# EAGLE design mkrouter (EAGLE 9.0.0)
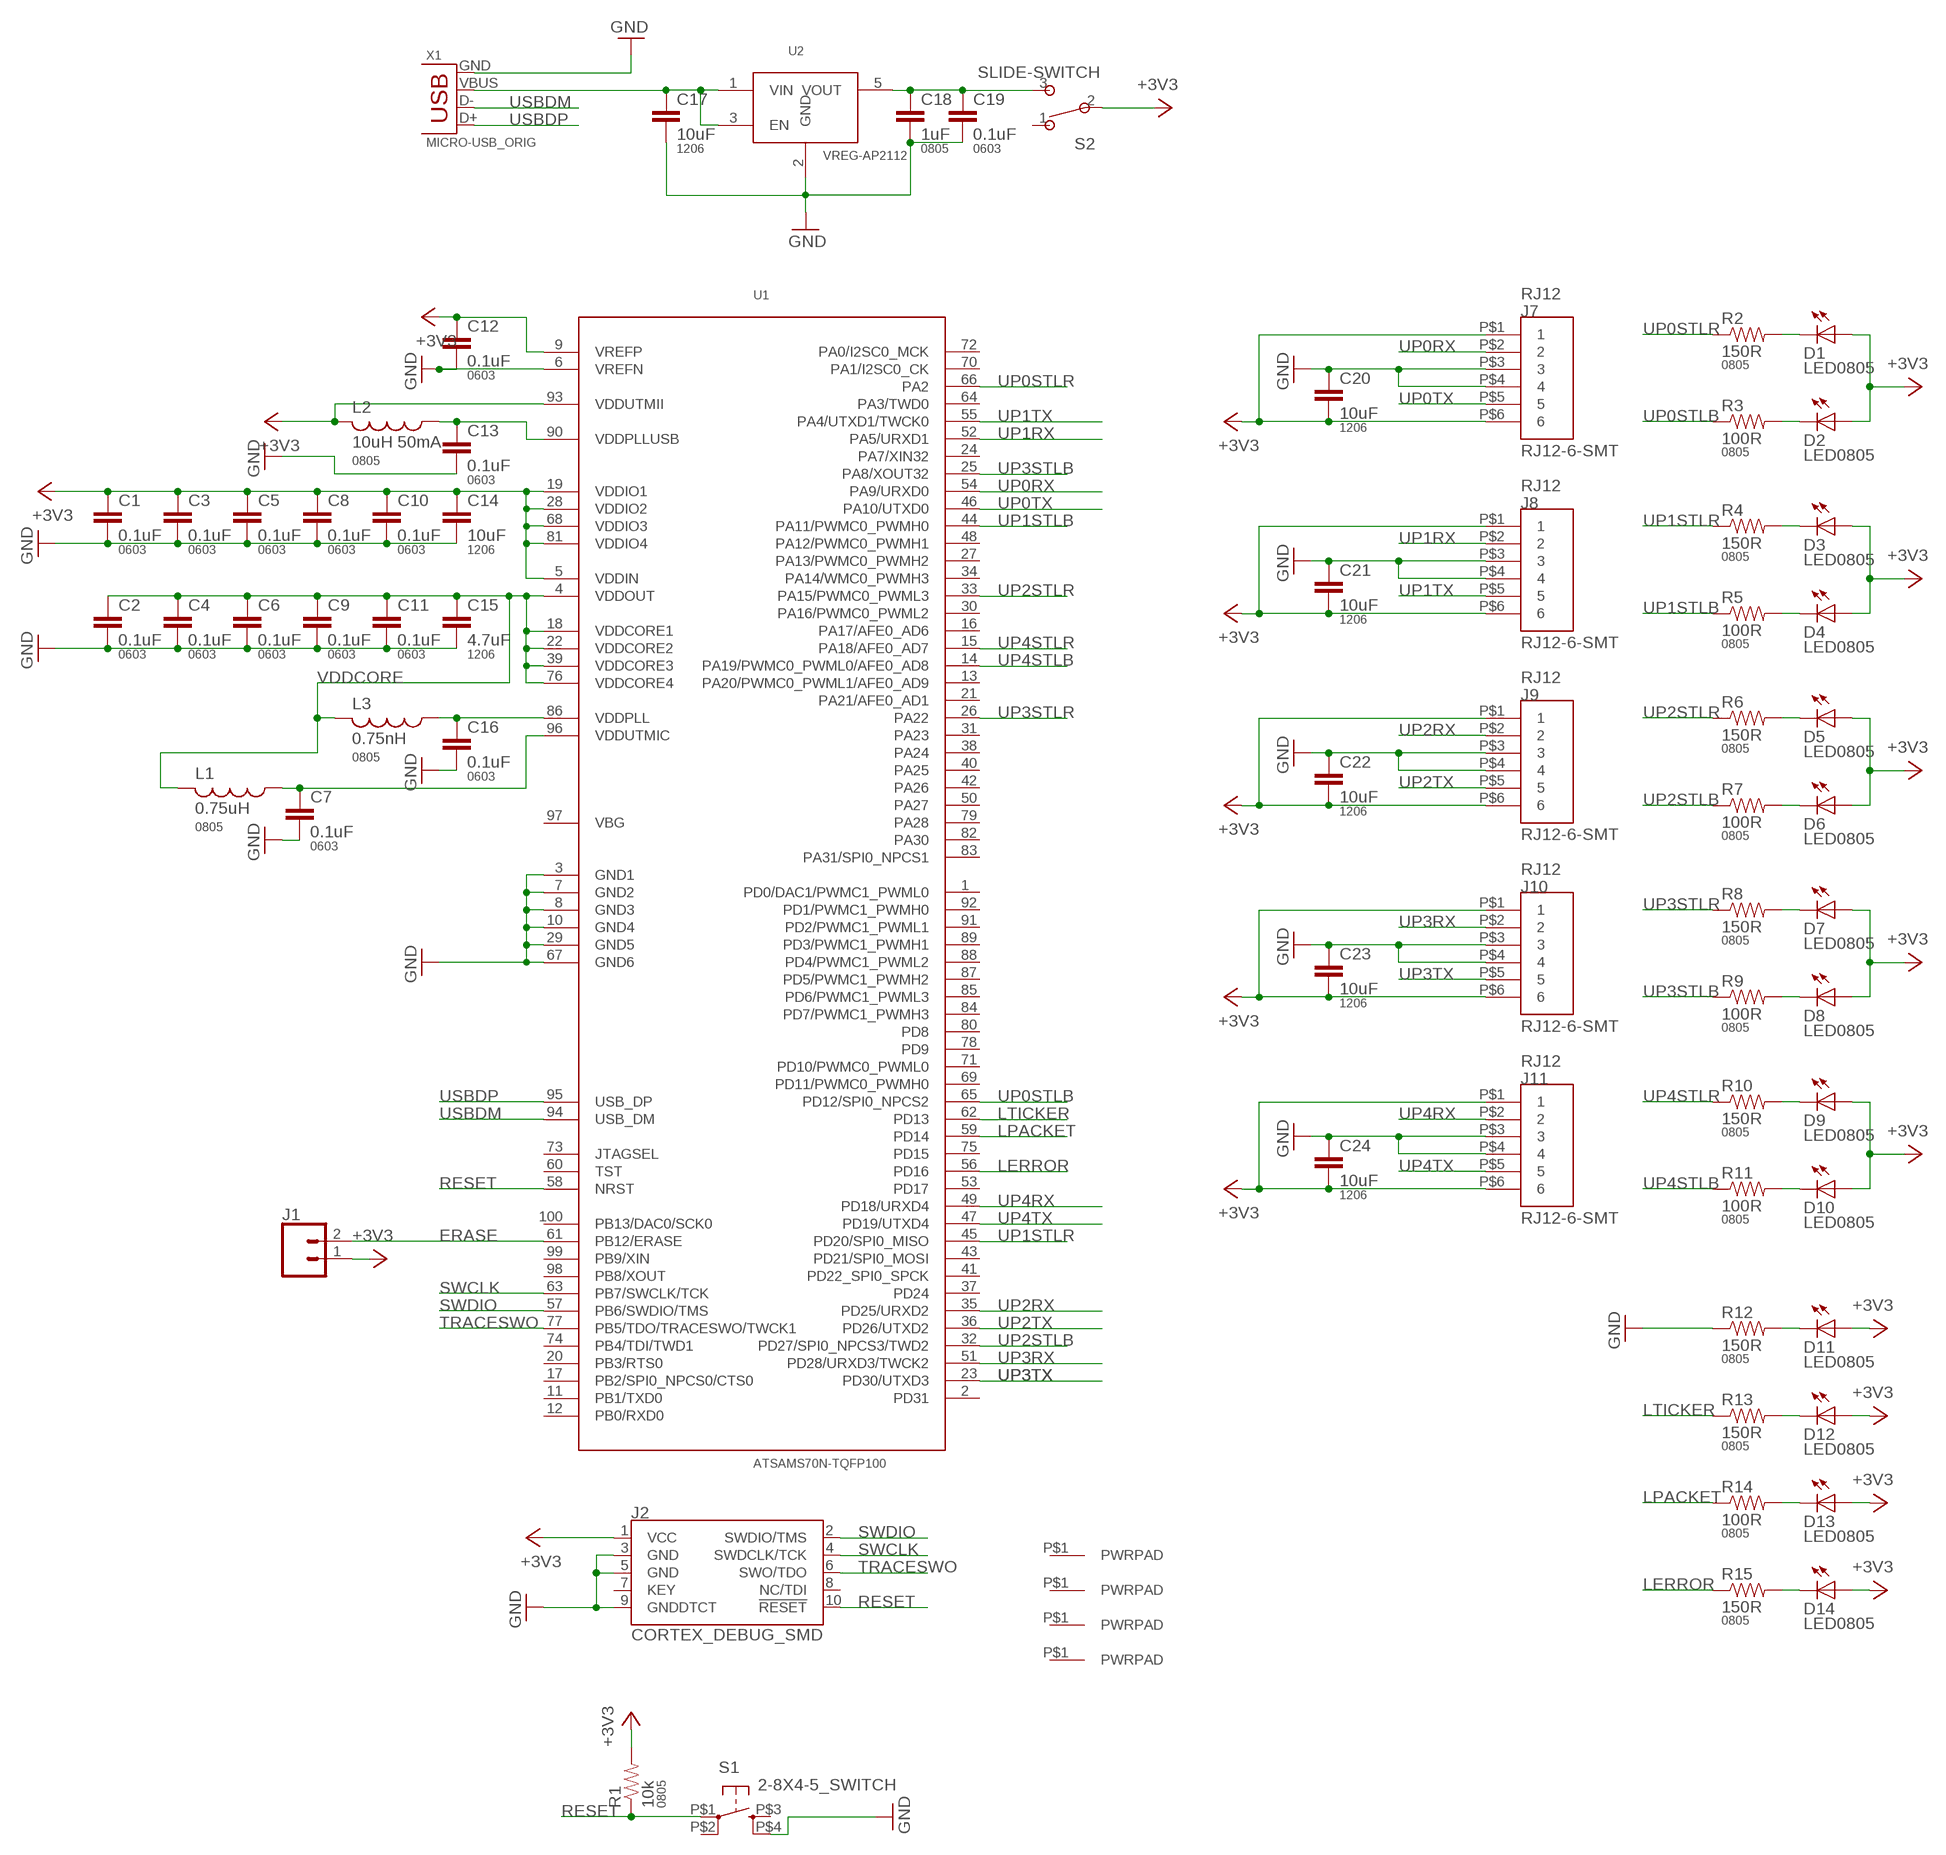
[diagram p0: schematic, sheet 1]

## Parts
C1  0.1uF  CAP0603-CAP  [0603-CAP]
C2  0.1uF  CAP0603-CAP  [0603-CAP]
C3  0.1uF  CAP0603-CAP  [0603-CAP]
C4  0.1uF  CAP0603-CAP  [0603-CAP]
C5  0.1uF  CAP0603-CAP  [0603-CAP]
C6  0.1uF  CAP0603-CAP  [0603-CAP]
C7  0.1uF  CAP0603-CAP  [0603-CAP]
C8  0.1uF  CAP0603-CAP  [0603-CAP]
C9  0.1uF  CAP0603-CAP  [0603-CAP]
C10  0.1uF  CAP0603-CAP  [0603-CAP]
C11  0.1uF  CAP0603-CAP  [0603-CAP]
C12  0.1uF  CAP0603-CAP  [0603-CAP]
C13  0.1uF  CAP0603-CAP  [0603-CAP]
C14  10uF  CAP1206  [1206]
C15  4.7uF  CAP1206  [1206]
C16  0.1uF  CAP0603-CAP  [0603-CAP]
C17  10uF  CAP1206  [1206]
C18  1uF  CAP0805  [0805]
C19  0.1uF  CAP0603-CAP  [0603-CAP]
C20  10uF  CAP1206  [1206]
C21  10uF  CAP1206  [1206]
C22  10uF  CAP1206  [1206]
C23  10uF  CAP1206  [1206]
C24  10uF  CAP1206  [1206]
D1  LED0805  [LED0805]
D2  LED0805  [LED0805]
D3  LED0805  [LED0805]
D4  LED0805  [LED0805]
D5  LED0805  [LED0805]
D6  LED0805  [LED0805]
D7  LED0805  [LED0805]
D8  LED0805  [LED0805]
D9  LED0805  [LED0805]
D10  LED0805  [LED0805]
D11  LED0805  [LED0805]
D12  LED0805  [LED0805]
D13  LED0805  [LED0805]
D14  LED0805  [LED0805]
J1  CONN_021X02_NO_SILK  [1X02_NO_SILK]
J2  CORTEX_DEBUG_SMD  [SAMTECH_FTSH-105-01]
J3  PWRPADM3  [PWRPAD_3-25MM]
J4  PWRPADM3  [PWRPAD_3-25MM]
J5  PWRPADM3  [PWRPAD_3-25MM]
J6  PWRPADM3  [PWRPAD_3-25MM]
J7  RJ12-6-SMT  [RJ12-6-SMT]
J8  RJ12-6-SMT  [RJ12-6-SMT]
J9  RJ12-6-SMT  [RJ12-6-SMT]
J10  RJ12-6-SMT  [RJ12-6-SMT]
J11  RJ12-6-SMT  [RJ12-6-SMT]
L1  0.75uH  INDUCTOR-0805  [0805]
L2  10uH 50mA  INDUCTOR-0805  [0805]
L3  0.75nH  INDUCTOR-0805  [0805]
R1  10k  RESISTOR0805-RES  [0805]
R2  150R  RESISTOR0805-RES  [0805]
R3  100R  RESISTOR0805-RES  [0805]
R4  150R  RESISTOR0805-RES  [0805]
R5  100R  RESISTOR0805-RES  [0805]
R6  150R  RESISTOR0805-RES  [0805]
R7  100R  RESISTOR0805-RES  [0805]
R8  150R  RESISTOR0805-RES  [0805]
R9  100R  RESISTOR0805-RES  [0805]
R10  150R  RESISTOR0805-RES  [0805]
R11  100R  RESISTOR0805-RES  [0805]
R12  150R  RESISTOR0805-RES  [0805]
R13  150R  RESISTOR0805-RES  [0805]
R14  100R  RESISTOR0805-RES  [0805]
R15  150R  RESISTOR0805-RES  [0805]
S1  2-8X4-5_SWITCH  [TACT-SWITCH-KMR6]
S2  SLIDE-SWITCH  [AYZ0102AGRLC]
U1  ATSAMS70N-TQFP100  [TQFP100-14X14]
U2  VREG-AP2112  [SOT23-5]
X1  MICRO-USB_ORIG  [DX4R005HJ5]

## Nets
+3V3: C1.1 C3.1 C5.1 C8.1 C10.1 C12.1 C14.1 C20.2 C21.2 C22.2 C23.2 C24.2 D1.1(A) D2.1(A) D3.1(A) D4.1(A) D5.1(A) D6.1(A) D7.1(A) D8.1(A) D9.1(A) D10.1(A) D11.1(A) D12.1(A) D13.1(A) D14.1(A) J1.1 J2.1(VCC) J7.P$1 J7.P$6 J8.P$1 J8.P$6 J9.P$1 J9.P$6 J10.P$1 J10.P$6 J11.P$1 J11.P$6 L2.2 R1.2 S2.2 U1.5(VDDIN) U1.9(VREFP) U1.19(VDDIO1) U1.28(VDDIO2) U1.68(VDDIO3) U1.81(VDDIO4) U1.93(VDDUTMII)
ERASE: J1.2 U1.61(PB12/ERASE)
GND: C1.2 C2.2 C3.2 C4.2 C5.2 C6.2 C7.2 C8.2 C9.2 C10.2 C11.2 C12.2 C13.2 C14.2 C15.2 C16.2 C17.2 C18.2 C19.2 C20.1 C21.1 C22.1 C23.1 C24.1 J2.3(GND) J2.5(GND) J2.9(GNDDTCT) J7.P$3 J7.P$4 J8.P$3 J8.P$4 J9.P$3 J9.P$4 J10.P$3 J10.P$4 J11.P$3 J11.P$4 R12.1 S1.P$4(S1) U1.3(GND1) U1.6(VREFN) U1.7(GND2) U1.8(GND3) U1.10(GND4) U1.29(GND5) U1.67(GND6) U2.2(GND) X1.GND
LERROR: R15.1 U1.56(PD16)
LPACKET: R14.1 U1.59(PD14)
LTICKER: R13.1 U1.62(PD13)
N$1: C16.1 L3.1 U1.86(VDDPLL)
N$2: D4.2(C) R5.2
N$3: C7.1 L1.1 U1.96(VDDUTMIC)
N$4: C17.1 U2.1(VIN) U2.3(EN) X1.VBUS
N$5: C13.1 L2.1 U1.90(VDDPLLUSB)
N$6: D2.2(C) R3.2
N$7: C18.1 C19.1 S2.3 U2.5(VOUT)
N$8: D1.2(C) R2.2
N$9: D3.2(C) R4.2
N$10: D6.2(C) R7.2
N$11: D5.2(C) R6.2
N$12: D8.2(C) R9.2
N$13: D7.2(C) R8.2
N$14: D10.2(C) R11.2
N$15: D9.2(C) R10.2
N$16: D13.2(C) R14.2
N$17: D14.2(C) R15.2
N$22: D12.2(C) R13.2
N$23: D11.2(C) R12.2
RESET: J2.10(!RESET) R1.1 S1.P$1(P) U1.58(NRST)
SWCLK: J2.4(SWDCLK/TCK) U1.63(PB7/SWCLK/TCK)
SWDIO: J2.2(SWDIO/TMS) U1.57(PB6/SWDIO/TMS)
TRACESWO: J2.6(SWO/TDO) U1.77(PB5/TDO/TRACESWO/TWCK1)
UP0RX: J7.P$2 U1.54(PA9/URXD0)
UP0STLB: R3.1 U1.65(PD12/SPI0_NPCS2)
UP0STLR: R2.1 U1.66(PA2)
UP0TX: J7.P$5 U1.46(PA10/UTXD0)
UP1RX: J8.P$2 U1.52(PA5/URXD1)
UP1STLB: R5.1 U1.44(PA11/PWMC0_PWMH0)
UP1STLR: R4.1 U1.45(PD20/SPI0_MISO)
UP1TX: J8.P$5 U1.55(PA4/UTXD1/TWCK0)
UP2RX: J9.P$2 U1.35(PD25/URXD2)
UP2STLB: R7.1 U1.32(PD27/SPI0_NPCS3/TWD2)
UP2STLR: R6.1 U1.33(PA15/PWMC0_PWML3)
UP2TX: J9.P$5 U1.36(PD26/UTXD2)
UP3RX: J10.P$2 U1.51(PD28/URXD3/TWCK2)
UP3STLB: R9.1 U1.25(PA8/XOUT32)
UP3STLR: R8.1 U1.26(PA22)
UP3TX: J10.P$5 U1.23(PD30/UTXD3)
UP4RX: J11.P$2 U1.49(PD18/URXD4)
UP4STLB: R11.1 U1.14(PA19/PWMC0_PWML0/AFE0_AD8)
UP4STLR: R10.1 U1.15(PA18/AFE0_AD7)
UP4TX: J11.P$5 U1.47(PD19/UTXD4)
USBDM: U1.94(USB_DM) X1.D-
USBDP: U1.95(USB_DP) X1.D+
VDDCORE: C2.1 C4.1 C6.1 C9.1 C11.1 C15.1 L1.2 L3.2 U1.4(VDDOUT) U1.18(VDDCORE1) U1.22(VDDCORE2) U1.39(VDDCORE3) U1.76(VDDCORE4)
Unconnected: J2.7(KEY) J2.8(NC/TDI) J3.P$1(PWRPAD) J4.P$1(PWRPAD) J5.P$1(PWRPAD) J6.P$1(PWRPAD) S1.P$2(P1) S1.P$3(S) S2.1 U1.1(PD0/DAC1/PWMC1_PWML0) U1.2(PD31) U1.11(PB1/TXD0) U1.12(PB0/RXD0) U1.13(PA20/PWMC0_PWML1/AFE0_AD9) U1.16(PA17/AFE0_AD6) U1.17(PB2/SPI0_NPCS0/CTS0) U1.20(PB3/RTS0) U1.21(PA21/AFE0_AD1) U1.24(PA7/XIN32) U1.27(PA13/PWMC0_PWMH2) U1.30(PA16/PWMC0_PWML2) U1.31(PA23) U1.34(PA14/WMC0_PWMH3) U1.37(PD24) U1.38(PA24) U1.40(PA25) U1.41(PD22_SPI0_SPCK) U1.42(PA26) U1.43(PD21/SPI0_MOSI) U1.48(PA12/PWMC0_PWMH1) U1.50(PA27) U1.53(PD17) U1.60(TST) U1.64(PA3/TWD0) U1.69(PD11/PWMC0_PWMH0) U1.70(PA1/I2SC0_CK) U1.71(PD10/PWMC0_PWML0) U1.72(PA0/I2SC0_MCK) U1.73(JTAGSEL) U1.74(PB4/TDI/TWD1) U1.75(PD15) U1.78(PD9) U1.79(PA28) U1.80(PD8) U1.82(PA30) U1.83(PA31/SPI0_NPCS1) U1.84(PD7/PWMC1_PWMH3) U1.85(PD6/PWMC1_PWML3) U1.87(PD5/PWMC1_PWMH2) U1.88(PD4/PWMC1_PWML2) U1.89(PD3/PWMC1_PWMH1) U1.91(PD2/PWMC1_PWML1) U1.92(PD1/PWMC1_PWMH0) U1.97(VBG) U1.98(PB8/XOUT) U1.99(PB9/XIN) U1.100(PB13/DAC0/SCK0)

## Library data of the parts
C1-C13 C16 C19 = borkedlabs-passives:CAP: Capacitor; PACKAGE: 0603
C14 C15 C17 C20-C24 = borkedlabs-passives:CAP: Capacitor; PACKAGE: 1206
C18 = borkedlabs-passives:CAP: Capacitor; PACKAGE: 0805
D1-D14 = lights:LED: LED
J1 = SparkFun-Connectors:CONN_02: Multi connection point. Often used as Generic Header-pin footprint for 0.1 inch spaced/style header connections
J2 = SparkFun-Connectors:CORTEX_DEBUG: Cortex Debug Connector - 10 pin Supports JTAG debug, Serial Wire debug, and Serial Wire Viewer. PTH and SMD connector options available. General Connector Information Products: PTH Connector -via Digi-Key SparkFun PSoc SparkFun T
J3-J6 = power:PWRPAD
J7-J11 = connector:RJ12-6-SMT
L1-L3 = borkedlabs-passives:INDUCTOR; PACKAGE: 0805
R1-R15 = borkedlabs-passives:RESISTOR: Resistor; PACKAGE: 0805
S1 = fab:2-8X4-5_SWITCH
S2 = fab:SLIDE-SWITCH: SMD slide-switch AYZ0102AGRLC as found in the fablab inventory. Includes the mounting holes. Made by Zaerc.
U1 = atsam:ATSAMS70N-TQFP100
U2 = power:VREG-AP2112
X1 = fab:MICRO-USB: SMD micro USB connector as found in the fablab inventory. Three footprint variants included: original, as described by manufacturer's datasheet for milling with the 1/100" bit for milling with the 1/64" bit Made by Zaerc.

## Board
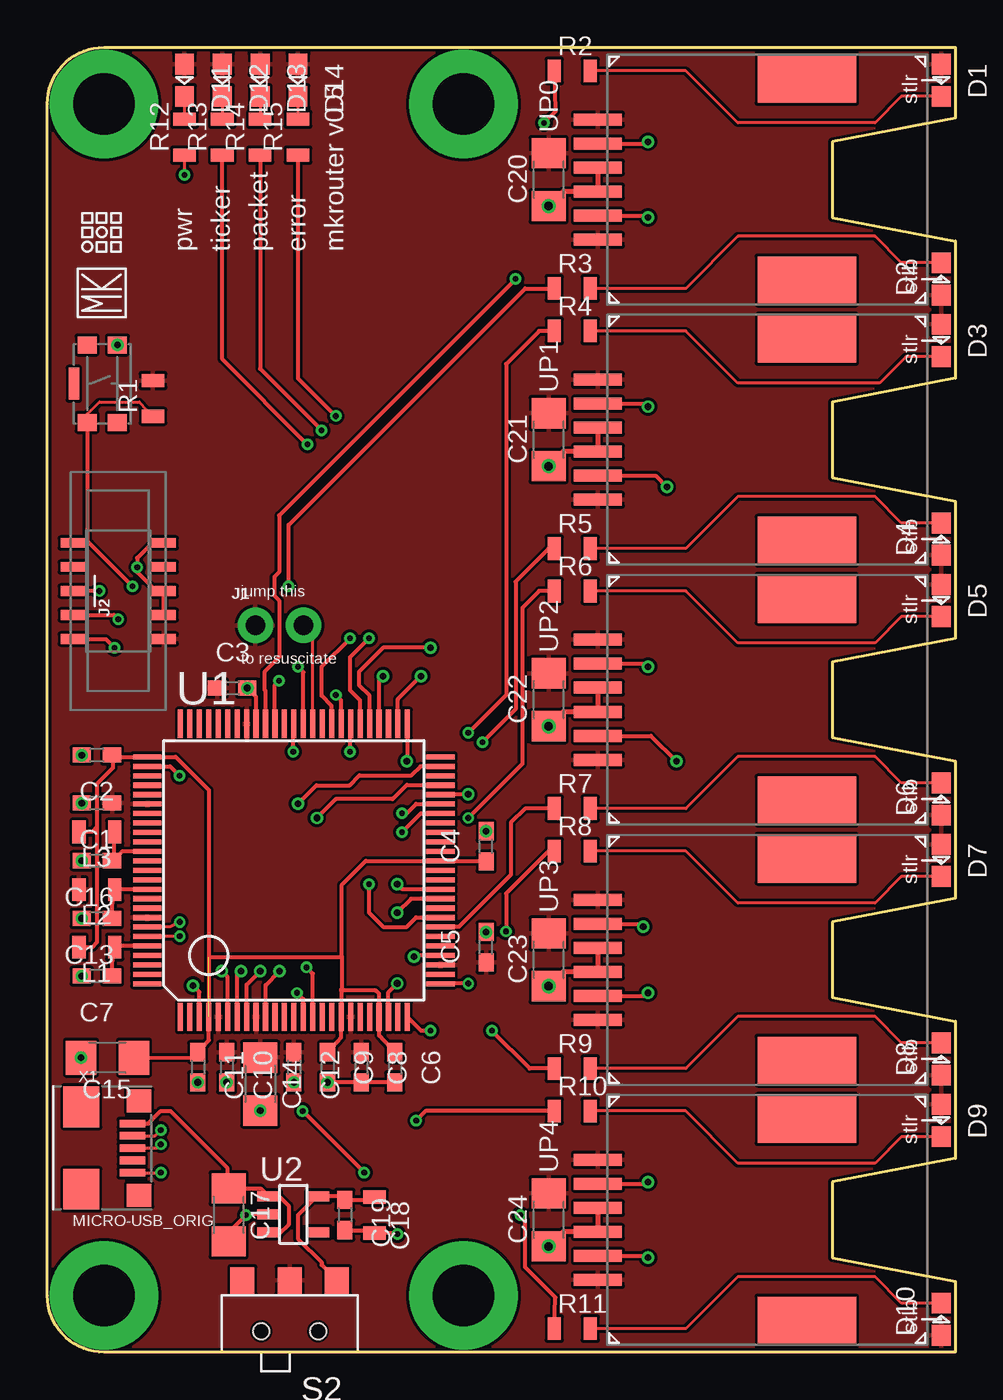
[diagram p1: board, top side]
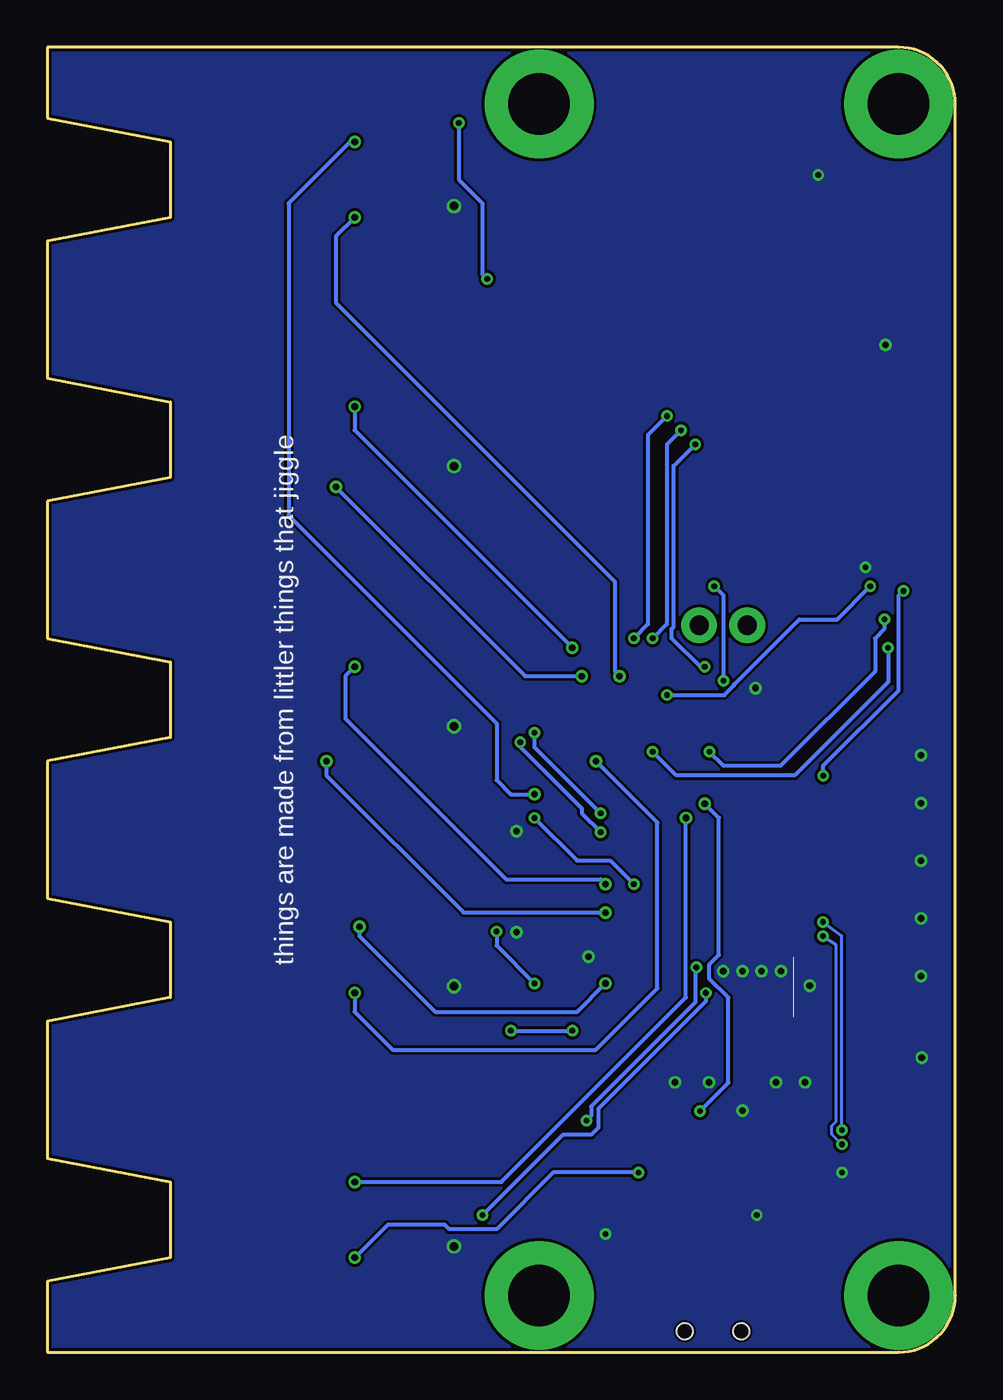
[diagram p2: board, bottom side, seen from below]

Size 48 x 69 mm. Coordinates in mm from the lower left corner, seen from the top.
Outline: 3,69 48,69 48,65.25 41.5,64 41.5,60 48,58.75 48,51.5 41.5,50.25 41.5,46.25 48,45 48,37.75 41.5,36.5 41.5,32.5 48,31.25 48,24 41.5,22.75 41.5,18.75 48,17.5 48,10.25 41.5,9 41.5,5 48,3.75 48,0 3,0 arc-90 0,3 0,66 arc-90 3,69
Copper layers (1*16): Top 0.035mm / dielectric 1.5mm / Bottom 0.035mm
Design rules "default *": minimum track width 6mil, minimum drill 0.3mm, track to track 6mil, track to pad 6mil, pad to pad 6mil, via to via 6mil, smd to smd 6mil, copper to edge 6mil, drill to drill 6mil, minimum pad ring 10mil, minimum via ring 6mil, stop-mask expansion 4mil, vias tented up to drill 20mil, thermal gap 6mil

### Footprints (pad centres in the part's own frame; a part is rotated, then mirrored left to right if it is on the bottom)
0603-CAP = smd 0.96 x 0.8: 1 -0.8,0; 2 0.8,0
1206 = smd 1.6 x 1.8: 1 -1.4,0; 2 1.4,0
0805 = smd 0.7 x 1.2: 1 -0.95,0; 2 0.95,0
LED0805 = smd 1.1 x 1: 1 -0.85,0; 2 0.85,0
1X02_NO_SILK = drill 1.016 pad 1.88: 1 0,0; 2 2.54,0
SAMTECH_FTSH-105-01 = smd 0.508 x 1.27: 1 -2.54,-2.413; 2 -2.54,2.413; 3 -1.27,-2.413; 4 -1.27,2.413; 5 0,-2.413; 6 0,2.413; 7 1.27,-2.413; 8 1.27,2.413; 9 2.54,-2.413; 10 2.54,2.413
PWRPAD_3-25MM = drill 3.25 pad 5.75: P$1 0,0
RJ12-6-SMT = smd 0.635 x 2.54: P$1 -3.175,17.399; P$2 -1.905,17.399; P$3 -0.635,17.399; P$4 0.635,17.399; P$5 1.905,17.399; P$6 3.175,17.399 | smd 2.54 x 5.207: P$7 -5.334,6.35; P$8 5.334,6.35
TACT-SWITCH-KMR6 = smd 0.9 x 1: P$1 -2.05,0.8; P$2 2.05,0.8; P$3 -2.05,-0.8; P$4 2.05,-0.8 | smd 1.7 x 0.55: P$5 0,1.5
AYZ0102AGRLC = smd 1.27 x 1.397: 1 2.5,-2.3; 2 0,-2.3; 3 -2.5,-2.3 | hole 0.85: -1.5,0.4; 1.5,0.4
TQFP100-14X14 = smd 0.27 x 1.5: 1 -6,-7.75; 2 -5.5,-7.75; 3 -5,-7.75; 4 -4.5,-7.75; 5 -4,-7.75; 6 -3.5,-7.75; 7 -3,-7.75; 8 -2.5,-7.75; 9 -2,-7.75; 10 -1.5,-7.75; 11 -1,-7.75; 12 -0.5,-7.75; 13 0,-7.75; 14 0.5,-7.75; 15 1,-7.75; 16 1.5,-7.75; 17 2,-7.75; 18 2.5,-7.75; 19 3,-7.75; 20 3.5,-7.75; 21 4,-7.75; 22 4.5,-7.75; 23 5,-7.75; 24 5.5,-7.75; 25 6,-7.75; 51 6,7.75; 52 5.5,7.75; 53 5,7.75; 54 4.5,7.75; 55 4,7.75; 56 3.5,7.75; 57 3,7.75; 58 2.5,7.75; 59 2,7.75; 60 1.5,7.75; 61 1,7.75; 62 0.5,7.75; 63 0,7.75; 64 -0.5,7.75; 65 -1,7.75; 66 -1.5,7.75; 67 -2,7.75; 68 -2.5,7.75; 69 -3,7.75; 70 -3.5,7.75; 71 -4,7.75; 72 -4.5,7.75; 73 -5,7.75; 74 -5.5,7.75; 75 -6,7.75 | smd 1.5 x 0.27: 26 7.75,-6; 27 7.75,-5.5; 28 7.75,-5; 29 7.75,-4.5; 30 7.75,-4; 31 7.75,-3.5; 32 7.75,-3; 33 7.75,-2.5; 34 7.75,-2; 35 7.75,-1.5; 36 7.75,-1; 37 7.75,-0.5; 38 7.75,0; 39 7.75,0.5; 40 7.75,1; 41 7.75,1.5; 42 7.75,2; 43 7.75,2.5; 44 7.75,3; 45 7.75,3.5; 46 7.75,4; 47 7.75,4.5; 48 7.75,5; 49 7.75,5.5; 50 7.75,6; 76 -7.75,6; 77 -7.75,5.5; 78 -7.75,5; 79 -7.75,4.5; 80 -7.75,4; 81 -7.75,3.5; 82 -7.75,3; 83 -7.75,2.5; 84 -7.75,2; 85 -7.75,1.5; 86 -7.75,1; 87 -7.75,0.5; 88 -7.75,0; 89 -7.75,-0.5; 90 -7.75,-1; 91 -7.75,-1.5; 92 -7.75,-2; 93 -7.75,-2.5; 94 -7.75,-3; 95 -7.75,-3.5; 96 -7.75,-4; 97 -7.75,-4.5; 98 -7.75,-5; 99 -7.75,-5.5; 100 -7.75,-6
SOT23-5 = smd 0.533 x 1.194: 1 -0.95,-1.306; 2 0,-1.306; 3 0.95,-1.306; 4 0.95,1.306; 5 -0.95,1.306
DX4R005HJ5 = smd 0.4 x 1.35: D+ 0,1.6; D- -0.65,1.6; GND 1.3,1.6; ID 0.65,1.6; VBUS -1.3,1.6 | smd 1.2 x 1.3: GND@1 -2.5,1.95; GND@2 2.5,1.95 | smd 2.15 x 1.9: GND@3 -2.175,-1.1; GND@4 2.175,-1.1

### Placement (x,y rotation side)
C1  2.62,29.04 180 top
C2  2.62,31.58 180 top
C3  9.77,35.12 0 top
C4  23.19,26.75 90 top
C5  23.19,21.42 90 top
C6  18.37,15.07 270 top
C7  2.62,19.89 180 top
C8  16.59,15.07 270 top
C9  14.81,15.07 270 top
C10  9.48,15.07 270 top
C11  7.95,15.07 270 top
C12  13.03,15.07 270 top
C13  2.62,22.94 180 top
C14  11.26,14.18 270 top
C15  3.18,15.57 180 top
C16  2.62,25.99 180 top
C17  9.58,7.26 270 top
C18  17.29,7.25 270 top
C19  15.72,7.26 270 top
C20  26.5,62 90 top
C21  26.5,48.25 90 top
C22  26.5,34.5 90 top
C23  26.5,20.75 90 top
C24  26.5,7 90 top
D1  47.25,67.25 270 top
D2  47.25,56.75 90 top
D3  47.25,53.5 270 top
D4  47.25,43 90 top
D5  47.25,39.75 270 top
D6  47.25,29.25 90 top
D7  47.25,26 270 top
D8  47.25,15.5 90 top
D9  47.25,12.25 270 top
D10  47.25,1.75 90 top
D11  7.25,67.25 270 top
D12  9.25,67.25 270 top
D13  11.25,67.25 270 top
D14  13.25,67.25 270 top
J1  11,38.43 0 top
J2  3.75,40.25 90 top
J3  22,66 0 top
J4  22,3 0 top
J5  3,3 0 top
J6  3,66 0 top
J7  46.5,62 90 top
J8  46.5,48.25 90 top
J9  46.5,34.5 90 top
J10  46.5,20.75 90 top
J11  46.5,7 90 top
L1  2.62,21.42 180 top
L2  2.62,24.46 180 top
L3  2.62,27.51 180 top
R1  5.58,50.43 90 top
R2  27.75,67.75 0 top
R3  27.75,56.25 0 top
R4  27.75,54 0 top
R5  27.75,42.5 0 top
R6  27.75,40.25 0 top
R7  27.75,28.75 0 top
R8  27.75,26.5 0 top
R9  27.75,15 0 top
R10  27.75,12.75 0 top
R11  27.75,1.25 0 top
R12  7.25,64.25 90 top
R13  9.25,64.25 90 top
R14  11.25,64.25 90 top
R15  13.25,64.25 90 top
S1  2.9,51.21 90 top
S2  12.81,1.5 180 top
U1  13.03,25.48 0 top
U2  13.01,7.29 270 top
U$1  [CBA-SILK-LOGO]  2.87,59.22 90 top
U$2  [MK-LOGO-SILK]  2.87,56.01 90 top
X1  2.9,10.8 270 top

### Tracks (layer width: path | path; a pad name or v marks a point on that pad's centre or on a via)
+3V3
  pour Top (rank 2): 0,69 0,0 48,0 48,69
ERASE
  Top 0.152: U1.61 14.03,37.94 J1.2
GND  (via drill 0.3, 0.35, 0.45)
  Top 0.152: X1.GND v6,9.5 | R12.1 v7.25,62.25
  Top 0.2: U2.2 10.54,7.29 v10.5,7.25
  Top 0.203: U1.3 8.03,19.05 v7.7,19.38 | U1.6 9.53,19.84 v9.22,20.15 | U1.7 10.03,19.94 v10.24,20.15 | U1.8 10.53,19.42 v11.26,20.15 | U1.10 11.53,19.41 v12.27,20.15 | U1.29 19.46,20.98 v19.38,20.91 | C6.2 C8.2 C9.2 | C17.2 9.58,6.33 v10.5,7.25 | C19.2 17.18,6.46 C18.2 18.4,6.35 v18.5,6.25 | J2.3 J2.5 5.75,40.25 4.75,41.25 v4.75,41.5 4.75,42 5.54,42.79 J2.9 | U1.67 11.03,34.66 C3.2
  Top 0.254: J7.P$4 J7.P$3 27.27,61.36 C20.1 | J8.P$4 J8.P$3 27.27,47.62 C21.1 | J9.P$4 J9.P$3 27.27,33.87 C22.1 | J10.P$4 J10.P$3 27.27,20.11 C23.1 | J11.P$4 J11.P$3 27.27,6.37 C24.1
  other vias: 1.82,31.58 1.82,29.04 1.82,25.99 1.82,22.94 1.82,19.89 10.57,35.12 1.78,15.57 7.95,14.27 9.48,14.27 11.26,12.78 13.03,14.27 14.81,14.27 23.19,22.22 23.19,27.55 3.7,53.26 26.5,60.6 26.5,46.85 26.5,33.1 26.5,19.35 26.5,5.6
  pour Bottom: 0,69 48,69 48,0 0,0
LERROR  (via drill 0.3)
  Top 0.203: R15.1 13.25,51.5 v15.25,49.5 | v17,37.75 16,36.75 16,35 16.53,34.47 U1.56
  Bottom 0.203: v15.25,49.5 16.25,48.5 16.25,38.5 v17,37.75
LPACKET  (via drill 0.3)
  Top 0.203: R14.1 11.25,52 v14.5,48.75 | v16,37.75 14.5,36.25 14.5,34.71 15.03,34.18 U1.59
  Bottom 0.203: v14.5,48.75 15.25,48 15.25,38.5 v16,37.75
LTICKER  (via drill 0.3)
  Top 0.203: U1.62 13.53,35.97 v13.25,36.25 | v13.75,48 9.25,52.5 R13.1
  Bottom 0.203: v13.25,36.25 13.5,36.25 15,37.75 15,38.25 14.89,38.35 14.89,46.86 v13.75,48
N$1
  Top 0.203: 3.52,26.04 L3.1 | 3.52,26.04 C16.1 | U1.86 3.96,26.48 3.52,26.04
N$2
  Top 0.152: D4.2 45.15,43.85 43.75,45.25 36.5,45.25 33.75,42.5 R5.2
N$3
  Top 0.203: U1.96 3.58,21.48 L1.1 3.47,21.37 C7.1
N$4
  Top 0.2: X1.VBUS 5.35,12.1 6,12.75 6.5,12.75 9.5,9.75 9.5,8.75 C17.1 11.28,8.66 U2.1 12.26,8.24 12.75,7.75 12.75,6.75 12.25,6.25 11.79,6.25 U2.3
N$5
  Top 0.203: U1.90 3.54,24.48 L2.1 3.47,24.41 C13.1
N$6
  Top 0.152: D2.2 45.15,57.6 43.75,59 36.5,59 33.75,56.25 R3.2
N$7
  Top 0.2: C18.1 17.2,8.06 C19.1 15.54,8.24 U2.5 14.24,8.24 13.25,7.25 13.25,6 14.5,4.75 14.5,4.61 S2.3
N$8
  Top 0.152: D1.2 45.15,66.4 43.75,65 36.5,65 33.75,67.75 R2.2
N$9
  Top 0.152: D3.2 45.4,52.65 44,51.25 36.5,51.25 33.75,54 R4.2
N$10
  Top 0.152: D6.2 45.15,30.1 43.75,31.5 36.5,31.5 33.75,28.75 R7.2
N$11
  Top 0.152: D5.2 45.15,38.9 43.75,37.5 36.5,37.5 33.75,40.25 R6.2
N$12
  Top 0.152: D8.2 45.15,16.35 43.75,17.75 36.5,17.75 33.75,15 R9.2
N$13
  Top 0.152: D7.2 45.15,25.15 43.75,23.75 36.5,23.75 33.75,26.5 R8.2
N$14
  Top 0.152: D10.2 45.15,2.6 43.75,4 36.5,4 33.75,1.25 R11.2
N$15
  Top 0.152: D9.2 45.15,11.4 43.75,10 36.5,10 33.75,12.75 R10.2
N$16
  Top 0.152: D13.2 R14.2
N$17
  Top 0.152: D14.2 R15.2
N$22
  Top 0.152: D12.2 R13.2
N$23
  Top 0.152: D11.2 R12.2
RESET  (via drill 0.3)
  Top 0.152: S1.P$1 2.1,49.6 2.75,50.25 4.86,50.25 R1.1
  Top 0.203: U1.58 15.53,34.47 v15.25,34.75 | 2.25,42.75 v4.5,40.5 | 2.25,42.75 1.38,42.75 J2.10 | S1.P$1 2.1,42.9 2.25,42.75
  Bottom 0.203: v15.25,34.75 12.21,34.75 11.69,35.27 11.69,35.31 8.25,38.75 6.25,38.75 v4.5,40.5
SWCLK  (via drill 0.3)
  Top 0.203: J2.4 3.52,38.98 v3.75,38.75 | v13,31.75 13,33.2 U1.63
  Bottom 0.203: v3.75,38.75 3.75,38.25 4.25,37.75 4.25,36 9.25,31 12.25,31 v13,31.75
SWDIO  (via drill 0.3)
  Top 0.203: J2.2 3.1,37.71 v3.56,37.25 | v16,31.75 16,33.2 U1.57
  Bottom 0.203: v3.56,37.25 3.56,35.44 8.5,30.5 14.75,30.5 v16,31.75
TRACESWO  (via drill 0.3)
  Top 0.203: U1.77 6.49,30.98 v6.99,30.49 | v2.75,40.25 J2.6
  Bottom 0.203: v6.99,30.49 6.99,31.01 3,35 3,40 v2.75,40.25
UP0RX  (via drill 0.35)
  Top 0.203: J7.P$2 31.66,60.09 v31.75,60 | U1.54 17.53,35.53 v17.75,35.75
  Bottom 0.203: v31.75,60 32.75,59 32.75,55.5 18,40.75 18,36 v17.75,35.75
UP0STLB  (via drill 0.3)
  Top 0.203: U1.65 12.03,35.28 v12.25,35.5 | v12.75,40.5 12.75,43.75 25.25,56.25 R3.1
  Bottom 0.203: v12.25,35.5 12.25,40 v12.75,40.5
UP0STLR  (via drill 0.3)
  Top 0.203: R2.1 26.85,65.6 v26.25,65 | v24.75,56.75 12.25,44.25 12.25,41.25 12,41 12,40 12.25,39.75 12.25,36.75 11.5,36 11.5,35 11.53,34.97 U1.66
  Bottom 0.203: v26.25,65 26.25,62 25,60.75 25,57 v24.75,56.75
UP0TX  (via drill 0.35)
  Top 0.203: J7.P$5 31.66,63.91 v31.75,64 | v22.25,29.5 20.8,29.5 U1.46
  Bottom 0.203: v31.75,64 32,64 35.25,60.75 35.25,44.25 24.25,33.25 24.25,30.25 23.5,29.5 v22.25,29.5
UP1RX  (via drill 0.35)
  Top 0.203: J8.P$2 32.16,46.34 v32.75,45.75 | U1.52 18.53,34.53 v19.75,35.75
  Bottom 0.203: v32.75,45.75 22.75,35.75 v19.75,35.75
UP1STLB  (via drill 0.3)
  Top 0.203: R5.1 26.5,42.5 24.75,40.75 24.75,34 v23,32.25 | v18.75,27.5 19.75,28.5 20.76,28.5 U1.44
  Bottom 0.203: v23,32.25 23,32 19.75,28.75 19.75,28.5 v18.75,27.5
UP1STLR  (via drill 0.3)
  Top 0.203: R4.1 26,54 24.25,52.25 24.25,34.75 v22.25,32.75 | v18.75,28.5 19,28.5 19.5,29 20.76,29 U1.45
  Bottom 0.203: v22.25,32.75 22.25,32 v18.75,28.5
UP1TX  (via drill 0.35)
  Top 0.203: J8.P$5 31.59,50.16 v31.75,50 | v20.25,37.25 17.75,37.25 16.5,36 16.5,35.25 17.03,34.72 U1.55
  Bottom 0.203: v31.75,50 31.75,48.75 v20.25,37.25
UP2RX  (via drill 0.35)
  Top 0.203: J9.P$2 31.91,32.59 v33.25,31.25 | U1.35 19.23,23.98 v18.5,23.25
  Bottom 0.203: v33.25,31.25 33.25,30.5 26,23.25 v18.5,23.25
UP2STLB
  Top 0.203: R7.1 25.25,28.75 24.5,28 24.5,25.25 21.75,22.5 20.8,22.5 U1.32
UP2STLR  (via drill 0.3)
  Top 0.203: R6.1 26,40.25 25.11,39.36 25.11,31.11 v22.25,28.25 | v17,24.75 17,23.25 17.75,22.5 19,22.5 19.5,23 20.76,23 U1.33
  Bottom 0.203: v22.25,28.25 20,26 18.25,26 v17,24.75
UP2TX  (via drill 0.35)
  Top 0.203: J9.P$5 31.59,36.41 v31.75,36.25 | U1.36 18.77,24.48 v18.5,24.75
  Bottom 0.203: v31.75,36.25 32.25,35.75 32.25,33.5 23.75,25 18.75,25 v18.5,24.75
UP3RX  (via drill 0.35)
  Top 0.203: J10.P$2 31.59,18.84 v31.75,19 | U1.51 19.03,31.28 v19,31.25
  Bottom 0.203: v31.75,19 31.75,18 29.75,16 19,16 15.75,19.25 15.75,28 v19,31.25
UP3STLB  (via drill 0.3)
  Top 0.203: R9.1 25.5,15 v23.5,17 | v20.25,17 19.76,17 U1.25
  Bottom 0.203: v23.5,17 v20.25,17
UP3STLR  (via drill 0.3)
  Top 0.203: R8.1 26.5,26.5 24.25,24.25 v24.25,22.25 | v22.25,19.5 20.8,19.5 U1.26
  Bottom 0.203: v24.25,22.25 24.25,21.5 v22.25,19.5
UP3TX  (via drill 0.35)
  Top 0.203: J10.P$5 31.34,22.66 v31.5,22.5 | U1.23 18.03,19.03 v18.5,19.5
  Bottom 0.203: v31.5,22.5 31.5,22 27.5,18 20,18 v18.5,19.5
UP4RX  (via drill 0.3, 0.35)
  Top 0.203: J11.P$2 31.66,5.1 v31.75,5 | U1.49 19.73,30.98 19.25,30.5 16.5,30.5 15.98,29.98 14.23,29.98 v13.25,29 | v16.75,9.5 v13.5,12.75
  Bottom 0.203: v13.25,29 12.5,28.25 12.5,21 13,20.5 13,19.75 12,18.75 12,14.25 v13.5,12.75 | v16.75,9.5 21.25,9.5 24.25,6.5 26.75,6.5 27,6.75 30,6.75 v31.75,5
UP4STLB  (via drill 0.3)
  Top 0.203: U1.14 13.53,18.66 v13.19,19 | R11.1 26.85,2.9 25.25,4.5 25.25,7 v25,7.25
  Bottom 0.203: v13.19,19 13.19,18.55 17.14,14.6 18.87,12.87 18.87,11.88 19.25,11.5 20.75,11.5 v25,7.25
UP4STLR  (via drill 0.3)
  Top 0.203: R10.1 20,12.75 v19.5,12.25 | U1.15 14.03,20.01 v13.69,20.35
  Bottom 0.203: v13.69,20.35 13.75,20.3 13.75,18.5 19.25,13 19.25,12.5 v19.5,12.25
UP4TX  (via drill 0.35)
  Top 0.203: J11.P$5 31.66,8.9 v31.75,9 | U1.47 20.76,30 19,30 18.25,29.25 15.25,29.25 v14.25,28.25
  Bottom 0.203: v31.75,9 24,9 14.25,18.75 v14.25,28.25
USBDM  (via drill 0.3)
  Top 0.152: X1.D- 5.7,11.45 v6,11.75 | v7,22.75 6.5,22.5 5.3,22.5 U1.94
  Bottom 0.152: v6,11.75 6,22 v7,22.75
USBDP  (via drill 0.3)
  Top 0.152: X1.D+ 5.8,10.8 v6,10.99 | v7,21.99 5.3,21.99 U1.95
  Bottom 0.152: v6,10.99 v6,11 6.53,11.53 6.53,11.97 6.3,12.2 6.3,21.55 v7,21.99
VDDCORE  (1 unrouted)
  Top 0.203: 2.62,27.77 2.62,30.05 3.47,30.9 C2.1 3.57,31.48 U1.76 6.78,31.48 8.53,29.73 U1.4 8.53,16.5 C11.1 7.62,15.58 C15.1 | 2.62,27.77 2.37,27.51 L3.2 | 2.62,27.77 2.62,21.67 2.37,21.42 L1.2 | C9.1 15.53,16.64 U1.18 15.53,19.13 | C6.1 17.53,16.75 U1.22 17.53,18.95 17.35,19.13 15.53,19.13 | 15.53,19.13 15.53,19.17 | 15.57,20.91 15.57,24.72 16.84,25.98 U1.39 23.11,25.98 C4.1 | 15.57,20.91 15.57,19.17 15.53,19.13 | 8.53,20.91 15.57,20.91

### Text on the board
tPlace: UP0 | pwr | ticker | packet | error | mkrouter v0.5 | UP1 | jump this | UP2 | to resuscitate | UP3 | UP4
bPlace: things are made from littler things that jiggle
